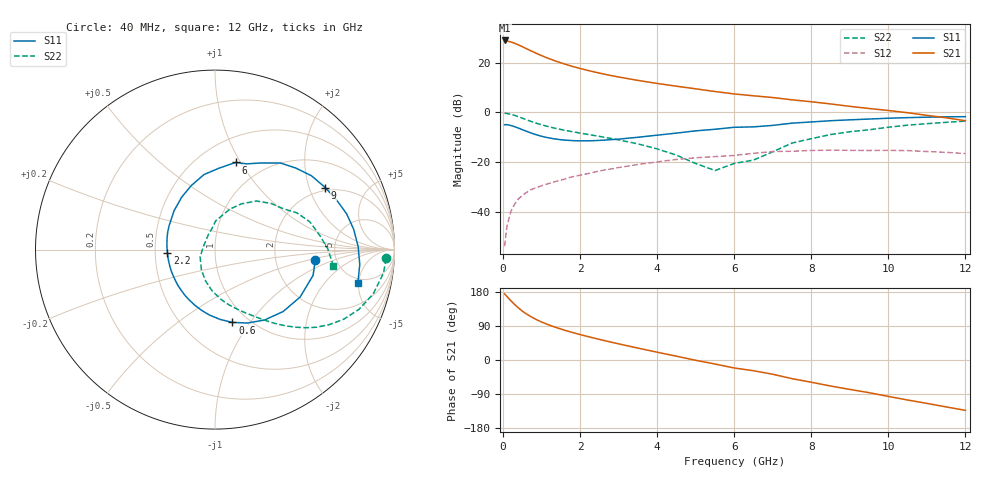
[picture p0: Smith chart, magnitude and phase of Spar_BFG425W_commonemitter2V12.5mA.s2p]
! Filename: 212bfg425.001
! BFG425W Field C1
! V1=8.516E-001V,V2=2.000E+000V, I1=1.713E-004A, I2=1.249E-002A
# GHz  S  MA  R 50
!  S11  S21  S12  S22
!Freq(GHz)  Mag  Ang  Mag  Ang  Mag  Ang  Mag  Ang
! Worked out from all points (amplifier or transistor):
!   44 points, 40 MHz to 12 GHz, reference 50 ohm
!   highest |S21| = 29.0 dB at 40 MHz (marker M1)
!   |S21| within 3 dB of that: start of sweep to 565.1 MHz
!   unconditionally stable (mu >= 1): 1.695 GHz to end of sweep
!   at 700 MHz: K = 0.60, MSG = 28.2 dB, |S12| = -31.4 dB
!   at 2.4 GHz: K = 1.13, MAG = 17.9 dB, |S12| = -24.0 dB
!   at 12 GHz: K = 1.37, MAG = 3.0 dB, |S12| = -16.7 dB
!   S11 on the Smith chart (normalised r, x): 40 MHz: 3.46, -0.57; 600 MHz: 0.84, -0.83; 2.2 GHz: 0.58, -0.02; 6 GHz: 0.74, +0.95; 9 GHz: 1.88, +2.58; 12 GHz: 4.38, -4.87
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0.04  0.562 -5.7  28.12 174.5  0.002 78.9  0.955 -2.9
0.1  0.565 -14.7  27.44 167.7  0.005 83.9  0.948 -7.9
0.2  0.543 -29.1  26.26 156.5  0.01 76.4  0.915 -15.7
0.3  0.513 -42.3  24.66 146.6  0.014 71.4  0.868 -22.6
0.4  0.48 -54.8  22.87 137.3  0.018 66.5  0.815 -28.5
0.5  0.447 -66.3  21.07 128.9  0.021 63.0  0.761 -33.3
0.6  0.417 -76.6  19.31 121.9  0.024 60.2  0.712 -37.4
0.8  0.366 -94.8  16.3 110.0  0.029 56.2  0.626 -43.7
0.9  0.346 -102.7  15.04 104.9  0.031 54.9  0.591 -46.3
1  0.329 -110.3  13.91 100.3  0.033 53.7  0.561 -48.5
1.2  0.304 -123.9  12.05 92.1  0.037 51.9  0.51 -52.5
1.6  0.275 -147.6  9.404 78.6  0.045 49.0  0.434 -59.2
2.2  0.266 -176.4  6.994 61.9  0.058 44.1  0.358 -69.0
3  0.288 152.7  5.152 42.6  0.077 35.8  0.278 -83.4
3.5  0.314 136.7  4.401 31.4  0.089 29.6  0.231 -93.9
4.5  0.381 110.1  3.362 10.0  0.112 15.5  0.137 -123.5
6  0.499 76.7  2.347 -21.1  0.135 -8.4  0.093 112.6
6.5  0.509 69.8  2.153 -28.3  0.149 -11.5  0.109 102.0
8.5  0.677 37.4  1.477 -68.7  0.173 -48.2  0.356 49.6
9  0.705 29.3  1.319 -77.6  0.171 -56.3  0.406 39.2
10.5  0.781 8.3  0.981 -105.6  0.169 -83.0  0.551 16.3
12  0.817 -13.1  0.677 -132.8  0.147 -112.6  0.665 -7.7
